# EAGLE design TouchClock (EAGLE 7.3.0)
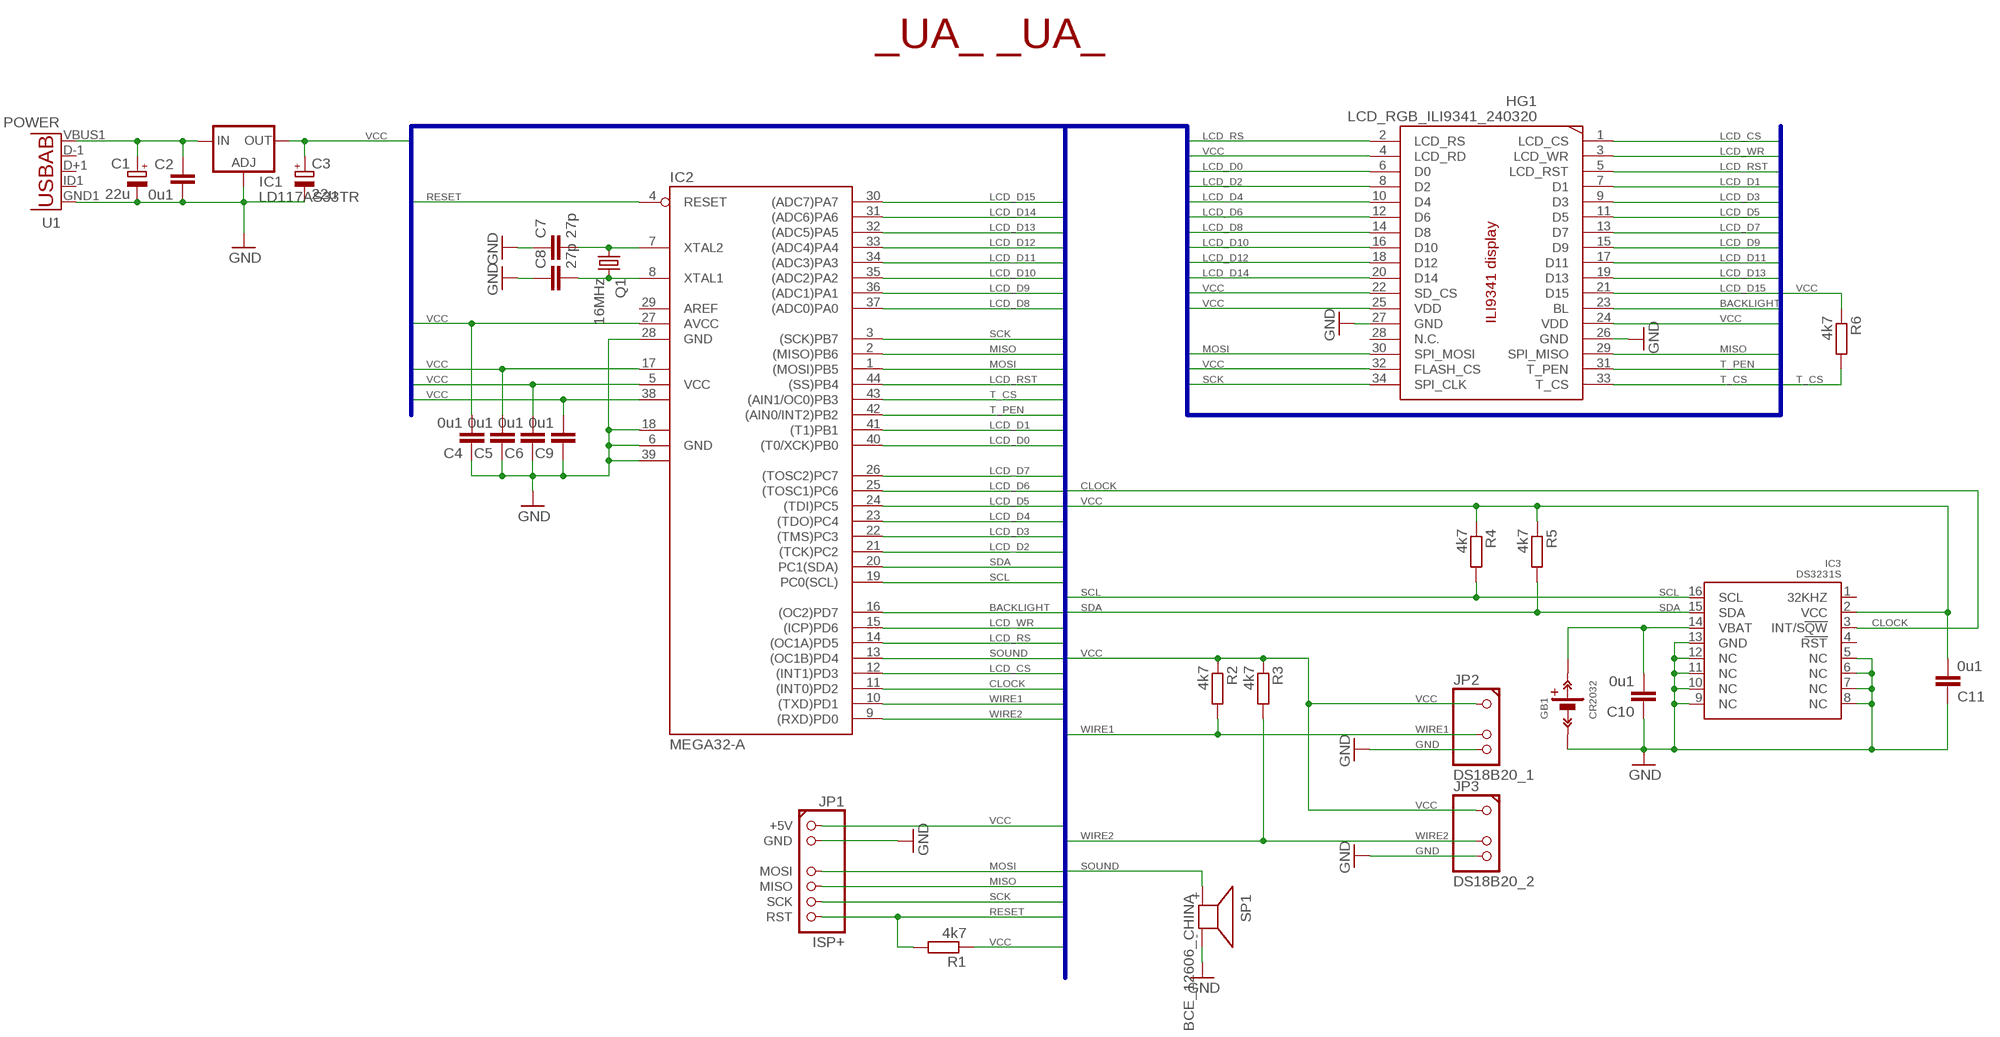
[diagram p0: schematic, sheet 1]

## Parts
C1  22u  CPOL-EUSMCB  [SMC_B]
C2  0u1  C-EUC1206T  [C1206T]
C3  22u  CPOL-EUSMCB  [SMC_B]
C4  0u1  C-EUC1206T  [C1206T]
C5  0u1  C-EUC1206T  [C1206T]
C6  0u1  C-EUC1206T  [C1206T]
C7  27p  C-EUC0805T  [C0805T]
C8  27p  C-EUC0805T  [C0805T]
C9  0u1  C-EUC1206T  [C1206T]
C10  0u1  C-EUC1206T  [C1206T]
C11  0u1  C-EUC1206T  [C1206T]
GB1  CR2032  CR2032_HOLDER/CH224  [CH224-2032]
HG1  LCD_RGB_ILI9341_240320  [2"4_320*240_ILI9341]
IC1  LD117AS33TR  [SOT223]
IC2  MEGA32-A  [TQFP44]
IC3  DS3231S  [SO16W]
JP1  ISP+  CONN1X7(2+4)_ISP+/R  [1X07_ISP+(ROUND)]
JP2  DS18B20_1  CONN1X4(1+2)/R90  [1X04ROUND/90(1+2)]
JP3  DS18B20_2  CONN1X4(1+2)/R90  [1X04ROUND/90(1+2)]
Q1  16MHz  CRYSTALHC49S  [HC49/S]
R1  4k7  R-EU_R0805T  [R0805T]
R2  4k7  R-EU_R0805T  [R0805T]
R3  4k7  R-EU_R0805T  [R0805T]
R4  4k7  R-EU_R0805T  [R0805T]
R5  4k7  R-EU_R0805T  [R0805T]
R6  4k7  R-EU_R0805T  [R0805T]
SP1  BCE_12606_CHINA  [BCE_12606_CHINA]
U1  POWER  USB5""  [USB-MICRO-SMD]
UA1  UA/MED  [UA_MED]
UA2  UA/SML  [UA_SMALL]

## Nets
BACKLIGHT: HG1.23(BL) IC2.16((OC2)PD7)
CLOCK: IC2.11((INT0)PD2) IC3.3(INT/SQW)
GND: C1.- C2.2 C3.- C4.1 C5.1 C6.1 C7.1 C8.1 C9.1 C10.1 C11.1 GB1.GB- HG1.26(GND) HG1.27(GND) IC1.1(ADJ) IC2.6(GND) IC2.18(GND1) IC2.28(GND) IC2.39(GND2) IC3.5(NC) IC3.6(NC) IC3.7(NC) IC3.8(NC) IC3.9(NC) IC3.10(NC) IC3.11(NC) IC3.12(NC) IC3.13(GND) JP1.GND JP2.4 JP3.4 SP1.- U1.GND1(GND)
LCD_CS: HG1.1(LCD_CS) IC2.12((INT1)PD3)
LCD_D0: HG1.6(D0) IC2.40((T0/XCK)PB0)
LCD_D1: HG1.7(D1) IC2.41((T1)PB1)
LCD_D2: HG1.8(D2) IC2.21((TCK)PC2)
LCD_D3: HG1.9(D3) IC2.22((TMS)PC3)
LCD_D4: HG1.10(D4) IC2.23((TDO)PC4)
LCD_D5: HG1.11(D5) IC2.24((TDI)PC5)
LCD_D6: HG1.12(D6) IC2.25((TOSC1)PC6)
LCD_D7: HG1.13(D7) IC2.26((TOSC2)PC7)
LCD_D8: HG1.14(D8) IC2.37((ADC0)PA0)
LCD_D9: HG1.15(D9) IC2.36((ADC1)PA1)
LCD_D10: HG1.16(D10) IC2.35((ADC2)PA2)
LCD_D11: HG1.17(D11) IC2.34((ADC3)PA3)
LCD_D12: HG1.18(D12) IC2.33((ADC4)PA4)
LCD_D13: HG1.19(D13) IC2.32((ADC5)PA5)
LCD_D14: HG1.20(D14) IC2.31((ADC6)PA6)
LCD_D15: HG1.21(D15) IC2.30((ADC7)PA7)
LCD_RS: HG1.2(LCD_RS) IC2.14((OC1A)PD5)
LCD_RST: HG1.5(LCD_RST) IC2.44((SS)PB4)
LCD_WR: HG1.3(LCD_WR) IC2.15((ICP)PD6)
MISO: HG1.29(SPI_MISO) IC2.2((MISO)PB6) JP1.MISO
MOSI: HG1.30(SPI_MOSI) IC2.1((MOSI)PB5) JP1.MOSI
N$1: C8.2 IC2.8(XTAL1) Q1.2
N$2: C7.2 IC2.7(XTAL2) Q1.1
N$5: C1.+ C2.1 IC1.3(IN) U1.VBUS1(VBUS)
RESET: IC2.4(RESET) JP1.RST R1.2
SCK: HG1.34(SPI_CLK) IC2.3((SCK)PB7) JP1.SCK
SCL: IC2.19(PC0(SCL)) IC3.16(SCL) R4.2
SDA: IC2.20(PC1(SDA)) IC3.15(SDA) R5.2
SOUND: IC2.13((OC1B)PD4) SP1.+
T_CS: HG1.33(T_CS) IC2.43((AIN1/OC0)PB3) R6.2
T_PEN: HG1.31(T_PEN) IC2.42((AIN0/INT2)PB2)
VBAT: C10.2 GB1.GB+ IC3.14(VBAT)
VCC: C3.+ C4.2 C5.2 C6.2 C9.2 C11.2 HG1.4(LCD_RD) HG1.22(SD_CS) HG1.24(VDD) HG1.25(VDD) HG1.32(FLASH_CS) IC1.4(OUT) IC2.5(VCC) IC2.17(VCC1) IC2.27(AVCC) IC2.38(VCC2) IC3.2(VCC) JP1.+5V JP2.1 JP3.1 R1.1 R2.1 R3.1 R4.1 R5.1 R6.1
WIRE1: IC2.10((TXD)PD1) JP2.3 R2.2
WIRE2: IC2.9((RXD)PD0) JP3.3 R3.2
Unconnected: HG1.28(N.C.) IC2.29(AREF) IC3.1(32KHZ) IC3.4(RST) U1.D+1(D+) U1.D-1(D-) U1.ID1(USBID)

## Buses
VCC,LCD_CS,LCD_WR,LCD_RST,LCD_RS,LCD_D[0..15],MISO,MOSI,SCK,T_PEN,T_CS,BACKLIGHT,RESET,SCL,SDA,WIRE1,WIRE2,CLOCK,SOUND

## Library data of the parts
C1 C3 = rcl:CPOL-EU: POLARIZED CAPACITOR, European symbol
C2 C4-C11 = rcl:C-EU: CAPACITOR, European symbol
GB1 = misc_passive_AL:CR2032_HOLDER: CR2032 Holder
HG1 = lcd-AL:LCD_RGB_ILI9341_240*320
IC1 = v-reg:LD117A?*: Low drop fixed and adjustable positive voltage regulators 1 A Source: http://www.st.com/stonline/products/literature/ds/7194/ld1117axx.pdf
IC2 = atmel:MEGA32: MICROCONTROLLER 32 Kbytes FLASH 2 Kbytes SRAM 1 Kbytes EEPROM USART 8-channel 10 bit ADC Source: www.atmel.com .. doc2503.pdf; MPN: ATMEGA32-16AU; OC_FARNELL: 9171274; OC_NEWARK: 69K6677
IC3 = misc-active-AL:DS3231S: TCXO Clock
JP1 = pinhead-AL:CONN1X7(2+4)_ISP+: PIN HEADER
JP2 JP3 = pinhead-AL:CONN1X4(1+2)
Q1 = crystal:CRYSTAL: CRYSTAL; OC_FARNELL: 1667008; OC_NEWARK: unknown
R1-R6 = rcl:R-EU_: RESISTOR, European symbol
SP1 = buzzer:BCE_12606_CHINA: BCE-12606
U1 = usb:USB5: This is a USB AB connector that is compatible with USB OTG. i.e. this connector can serve as a host or device
UA1 UA2 = misc_passive_AL:UA

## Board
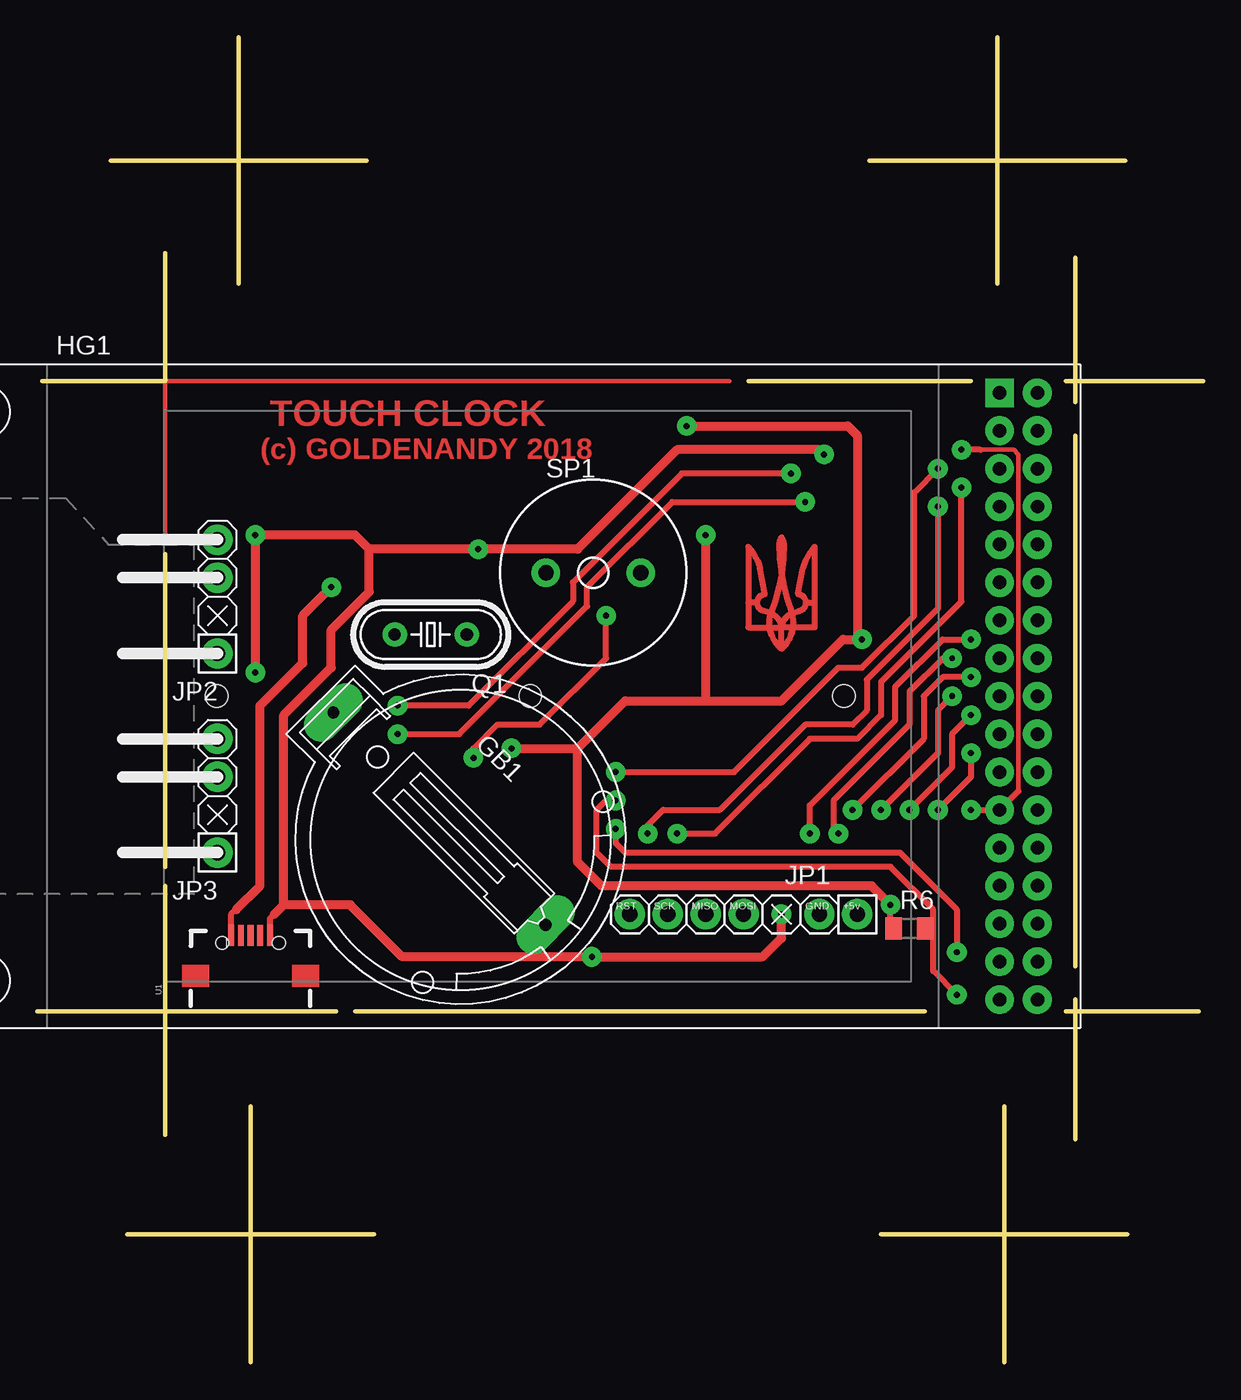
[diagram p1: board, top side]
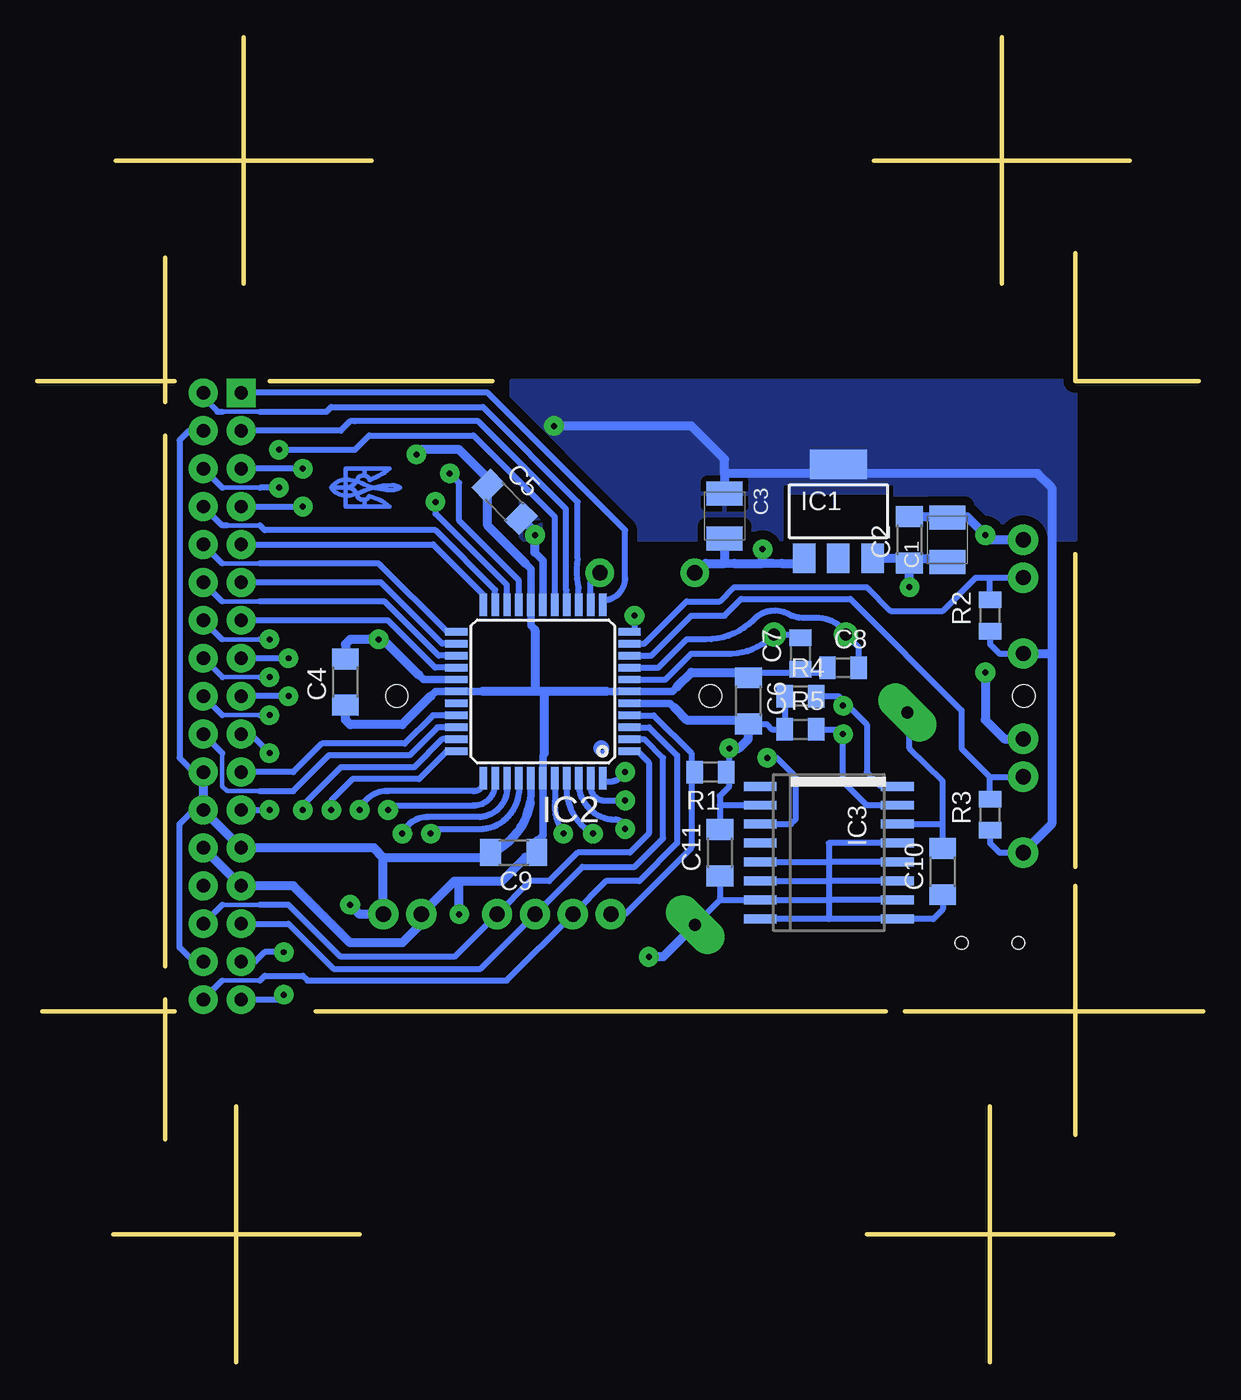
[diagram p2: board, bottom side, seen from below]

Size 78.11 x 88.74 mm. Coordinates in mm from the lower left corner, seen from the top.
Outline: 34 segments
Copper layers (1*16): Top 0.035mm / dielectric 1.5mm / Bottom 0.035mm
Design rules "default": minimum track width 12mil, minimum drill 10mil, track to track 10mil, track to pad 10mil, pad to pad 10mil, via to via 10mil, smd to smd 8mil, copper to edge 25mil, drill to drill 40mil, minimum pad ring 16mil, minimum via ring 18mil, stop-mask expansion 4mil, vias tented up to drill 0mil, thermal gap 16mil
Holes 1.5 mm at 54.02,44.61 33.02,44.61 12.02,44.61

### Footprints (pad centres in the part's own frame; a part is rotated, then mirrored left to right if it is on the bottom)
SMC_B = smd 1.6 x 2.4: + -1.5,0; - 1.5,0
C1206T = smd 1.4 x 1.8: 1 -1.55,0; 2 1.55,0
C0805T = smd 1.1 x 1.5: 1 -1.05,0; 2 1.05,0
CH224-2032 = drill 0.8 pad 2.3 long: GB+ -12.05,0; GB- 8.05,0
2"4_320*240_ILI9341 = drill 0.9 pad 1.93 square: 1 32.703,20.32 | drill 0.9 pad 1.93: 2 35.242,20.32; 3 32.703,17.78; 4 35.242,17.78; 5 32.703,15.24; 6 35.242,15.24; 7 32.703,12.7; 8 35.242,12.7; 9 32.703,10.16; 10 35.242,10.16; 11 32.703,7.62; 12 35.242,7.62; 13 32.703,5.08; 14 35.242,5.08; 15 32.703,2.54; 16 35.242,2.54; 17 32.703,0; 18 35.242,0; 19 32.703,-2.54; 20 35.242,-2.54; 21 32.703,-5.08; 22 35.242,-5.08; 23 32.703,-7.62; 24 35.242,-7.62; 25 32.703,-10.16; 26 35.242,-10.16; 27 32.703,-12.7; 28 35.242,-12.7; 29 32.703,-15.24; 30 35.242,-15.24; 31 32.703,-17.78; 32 35.242,-17.78; 33 32.703,-20.32; 34 35.242,-20.32
SOT223 = smd 1.5 x 2: 1 -2.3,-3.15; 2 0,-3.15; 3 2.3,-3.15 | smd 3.8 x 2: 4 0,3.15
TQFP44 = smd 1.5 x 0.5: 1 -5.8,4; 2 -5.8,3.2; 3 -5.8,2.4; 4 -5.8,1.6; 5 -5.8,0.8; 6 -5.8,0; 7 -5.8,-0.8; 8 -5.8,-1.6; 9 -5.8,-2.4; 10 -5.8,-3.2; 11 -5.8,-4; 23 5.8,-4; 24 5.8,-3.2; 25 5.8,-2.4; 26 5.8,-1.6; 27 5.8,-0.8; 28 5.8,0; 29 5.8,0.8; 30 5.8,1.6; 31 5.8,2.4; 32 5.8,3.2; 33 5.8,4 | smd 0.5 x 1.5: 12 -4,-5.8; 13 -3.2,-5.8; 14 -2.4,-5.8; 15 -1.6,-5.8; 16 -0.8,-5.8; 17 0,-5.8; 18 0.8,-5.8; 19 1.6,-5.8; 20 2.4,-5.8; 21 3.2,-5.8; 22 4,-5.8; 34 4,5.8; 35 3.2,5.8; 36 2.4,5.8; 37 1.6,5.8; 38 0.8,5.8; 39 0,5.8; 40 -0.8,5.8; 41 -1.6,5.8; 42 -2.4,5.8; 43 -3.2,5.8; 44 -4,5.8
SO16W = smd 0.6 x 2.2: 1 -4.445,-4.6; 2 -3.175,-4.6; 3 -1.905,-4.6; 4 -0.635,-4.6; 5 0.635,-4.6; 6 1.905,-4.6; 7 3.175,-4.6; 8 4.445,-4.6; 9 4.445,4.6; 10 3.175,4.6; 11 1.905,4.6; 12 0.635,4.6; 13 -0.635,4.6; 14 -1.905,4.6; 15 -3.175,4.6; 16 -4.445,4.6
1X07_ISP+(ROUND) = drill 1.016 pad 2.032: +5V -7.62,0; GND -5.08,0; MISO 2.54,0; MOSI 0,0; RST 7.62,0; SCK 5.08,0
1X04ROUND/90(1+2) = drill 1.016 pad 2.032: 1 -3.81,0; 3 1.27,0; 4 3.81,0
HC49/S = drill 0.813: 1 -2.413,0; 2 2.413,0
R0805T = smd 1.1 x 1.5: 1 -1.05,0; 2 1.05,0
BCE_12606_CHINA = drill 1.016 pad 1.905: + 3.175,0; - -3.175,0
USB-MICRO-SMD = smd 1.4 x 0.4: D+1 2.7,0; D-1 2.7,0.65; GND1 2.7,-1.3; ID1 2.7,-0.65; VBUS1 2.7,1.3 | hole 0.85: 2.2,1.9; 2.2,-1.9

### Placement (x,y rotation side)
C1  17.14,55.09 90 bottom
C2  19.69,55.09 90 bottom
C3  32.07,56.67 270 bottom
C4  57.47,45.56 90 bottom
C5  46.8,57.63 315 bottom
C6  30.48,44.29 270 bottom
C7  26.99,47.47 90 bottom
C8  24.13,46.51 0 bottom
C9  46.2,34.13 180 bottom
C10  17.46,32.86 90 bottom
C11  32.38,34.13 90 bottom
GB1  28.35,34.99 315 top
HG1  31.75,44.61 0 top
IC1  24.45,56.99 0 bottom
IC2  44.24,44.93 180 bottom
IC3  25.08,34.13 270 bottom
JP1  47.31,30 180 top
JP2  12.06,51.28 90 top
JP3  12.06,37.94 90 top
Q1  26.35,48.74 180 top
R1  33.02,39.53 180 bottom
R2  14.29,50.01 90 bottom
R3  14.29,36.67 90 bottom
R4  26.99,44.61 0 bottom
R5  26.99,42.39 0 bottom
R6  58.42,29.05 0 top
SP1  37.24,52.88 0 top
U1  14.29,25.88 90 top
UA1  49.85,51.28 0 top
UA2  56.52,58.58 270 bottom

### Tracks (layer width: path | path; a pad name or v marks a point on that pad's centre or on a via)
BACKLIGHT  (via drill 0.4)
  Top 0.305: 65.72,38.26 65.72,60.8 65.41,61.12 63.18,61.12
  Top 0.406: v62.55,36.99 HG1.23 65.72,38.26 | 63.18,61.12 v61.91,61.12
  Bottom 0.406: HG1.23 v62.55,36.99 | v61.91,61.12 56.83,61.12 55.88,62.07 48.9,62.07 43.44,56.62 IC2.16
CLOCK  (via drill 0.4)
  Top 0.406: v29.21,40.48 29.21,41.12 30.8,42.7 33.66,42.7 38.1,47.15 v38.1,50.01
  Bottom 0.406: IC3.3 27.62,36.04 27.3,36.35 27.3,39.21 28.58,40.48 v29.21,40.48 | v38.1,50.01 38.1,49.05 38.23,48.93 IC2.11
GND  (via drill 0.4)
  Top 0.406: U1.GND1 15.59,29.72 15.87,30
  Top 0.61: v49.85,30 49.85,28.42 48.58,27.15 v37.15,27.15 24.45,27.15 20.95,30.64 16.51,30.64 | 15.87,30 16.51,30.64 | 16.51,30.64 16.51,43.34 19.69,46.51 19.69,49.05 22.23,51.59 22.23,54.45 | v52.7,60.8 52.39,61.12 42.86,61.12 36.2,54.45 v29.53,54.45 22.23,54.45 | 22.23,54.45 21.27,55.4 v14.6,55.4 v14.6,46.2
  Bottom 0.406: 40.01,44.93 | 48.26,44.93 | C6.1 30.52,46.2 26.99,46.2 | 26.99,46.2 25.5,46.2 C8.1 | C7.1 26.99,46.2 | 25.08,29.69 IC3.9 18.1,29.69 17.46,30.32 C10.1 | 25.08,29.69 IC3.8 | IC3.10 25.08,30.96 | 25.08,30.96 25.08,29.69 | IC3.11 25.08,32.23 | 25.08,32.23 25.08,30.96 | IC3.12 25.08,33.5 | 25.08,33.5 25.08,32.23 | IC3.13 25.08,34.77 25.08,33.5 | 25.08,30.96 IC3.7 32.38,30.96 | IC3.6 25.08,32.23 | IC3.5 25.08,33.5 | GB1.GB- | GB1.GB- 32.38,30.96 | C11.1 32.38,30.96
  Bottom 0.508: 44.13,40.8 44.24,40.59 IC2.39 44.24,35.29 44.61,34.92 | 40.01,44.93 IC2.6 35.56,44.93 35.24,45.24 | 48.26,44.93 IC2.28 51.44,44.93 51.75,44.61 | 44.77,49.05 45.04,49.33 IC2.18 45.04,53.14 45.4,53.5
  Bottom 0.61: HG1.26 HG1.27 60.96,31.91 57.15,28.1 53.66,28.1 52.39,29.37 JP1.GND 50.17,32.23 49.85,32.23 | 44.77,49.05 44.77,44.93 | 44.77,44.93 48.26,44.93 | 40.01,44.93 44.13,44.93 | 44.13,44.93 44.77,44.93 | 44.13,40.8 44.13,44.93 | 35.24,45.24 34.29,46.2 30.52,46.2 | 45.4,53.5 47.94,56.04 47.94,58.68 C5.1 47.9,59.17 49.85,61.12 52.39,61.12 v52.7,60.8 | 44.61,34.92 44.77,34.77 44.77,33.81 | 44.77,33.81 45.4,33.81 46.99,32.23 49.85,32.23 | C9.1 44.77,33.81 | v49.85,30 49.85,32.23 | GB1.GB- | GB1.GB- 36.2,27.15 v37.15,27.15 | SP1.- 33.34,53.5 32.08,53.5 32.07,53.51 | C3.- 32.07,53.51 | 32.07,53.51 31.43,53.5 29.55,53.5 29.53,53.51 | 29.53,53.51 28.88,53.51 28.26,53.5 26.77,53.5 IC1.1 | 29.53,53.51 29.53,54.13 v29.53,54.45 | JP2.4 14.29,55.09 v14.6,55.4 15.84,56.64 17.14,56.64 | v14.6,46.2 14.6,43.02 13.33,41.75 JP3.4 | C2.2 17.14,56.64 | C1.- 17.14,56.64 | 51.75,44.61 53.66,42.7 57.15,42.7 57.47,43.02 C4.1
LCD_CS
  Bottom 0.406: HG1.1 47.94,64.93 38.73,55.72 38.73,52.55 arc93 40.24,51.04 IC2.12
LCD_D0  (via drill 0.4)
  Top 0.406: v42.86,35.4 45.4,35.4 51.75,41.75 54.93,41.75 56.52,43.34 56.52,45.56 61.91,50.96 v61.91,58.58
  Bottom 0.305: 63.18,58.58 65.72,58.58
  Bottom 0.406: IC2.40 43.44,37.57 arc-38 v42.86,35.4 | v61.91,58.58 63.18,58.58 | 65.72,58.58 HG1.6
LCD_D1  (via drill 0.4)
  Top 0.406: v40.88,35.4 40.88,35.96 41.91,36.99 45.72,36.99 51.44,42.7 54.61,42.7 55.56,43.66 55.56,45.72 60.33,50.48 v60.33,57.31
  Bottom 0.406: IC2.41 42.64,38.04 arc-54 v40.88,35.4 | HG1.7 v60.33,57.31
LCD_D2
  Bottom 0.305: 63.18,56.04 65.41,56.04
  Bottom 0.406: IC2.21 47.44,51.73 51.44,55.72 62.86,55.72 63.18,56.04 | 65.41,56.04 65.72,56.04 HG1.8
LCD_D3
  Bottom 0.406: HG1.9 51.59,54.77 48.24,51.42 IC2.22
LCD_D4
  Bottom 0.305: 65.72,53.5 63.18,53.5
  Bottom 0.406: HG1.10 65.72,53.5 | IC2.23 50.67,48.93 55.25,53.5 63.18,53.5
LCD_D5
  Bottom 0.406: IC2.24 50.98,48.13 55.09,52.23 HG1.11
LCD_D6
  Bottom 0.305: 65.72,50.96 63.18,50.96
  Bottom 0.406: HG1.12 65.72,50.96 | IC2.25 51.22,47.33 54.85,50.96 63.18,50.96
LCD_D7
  Bottom 0.406: IC2.26 51.45,46.53 54.61,49.69 HG1.13
LCD_D8  (via drill 0.4)
  Top 0.406: v51.75,35.4 51.75,37.31 57.47,43.02 57.47,45.24 60.64,48.42 v62.55,48.42
  Bottom 0.305: 65.72,48.42 63.18,48.42
  Bottom 0.406: HG1.14 65.72,48.42 | 63.18,48.42 v62.55,48.42 | IC2.37 45.84,38.14 arc79 48.26,35.72 51.44,35.72 v51.75,35.4
LCD_D9  (via drill 0.4)
  Top 0.406: v61.28,47.15 60.64,47.15 58.42,44.93 58.42,42.7 53.34,37.62 53.34,35.72 v53.66,35.4
  Bottom 0.406: IC2.36 46.64,38.29 arc79 48.42,36.51 51.91,36.51 arc-67 v53.66,35.4 | v61.28,47.15 HG1.15
LCD_D10  (via drill 0.4)
  Top 0.406: v62.55,45.88 60.64,45.88 59.37,44.61 59.37,41.75 v54.61,36.99
  Bottom 0.305: 65.72,45.88 63.18,45.88
  Bottom 0.406: HG1.16 65.72,45.88 | 63.18,45.88 v62.55,45.88 | v54.61,36.99 54.29,37.31 48.9,37.31 arc-96 47.44,38.76 IC2.35
LCD_D11  (via drill 0.4)
  Top 0.406: v61.28,44.61 60.33,43.66 60.33,40.8 v56.52,36.99
  Bottom 0.406: IC2.34 48.24,38.91 arc104 48.9,38.26 54.61,38.26 arc-70 v56.52,36.99 | v61.28,44.61 HG1.17
LCD_D12  (via drill 0.4)
  Top 0.406: v62.55,43.34 61.28,42.07 61.28,39.85 v58.42,36.99
  Bottom 0.305: 65.72,43.34 63.18,43.34
  Bottom 0.406: HG1.18 65.72,43.34 | 63.18,43.34 v62.55,43.34 | IC2.33 50.67,40.93 52.55,39.05 56.99,39.05 58.42,37.62 v58.42,36.99
LCD_D13  (via drill 0.4)
  Top 0.406: v62.55,40.8 62.55,39.21 v60.33,36.99
  Bottom 0.406: v60.33,36.99 60.33,37.31 57.78,39.85 52.86,39.85 50.98,41.73 IC2.32 | v62.55,40.8 63.82,42.07 HG1.19
LCD_D14
  Bottom 0.305: 65.72,40.8 65.72,38.58 65.41,38.26 63.18,38.26
  Bottom 0.406: HG1.20 65.72,40.8 | 63.18,38.26 60.96,38.26 58.58,40.64 53.18,40.64 51.3,42.53 IC2.31
LCD_D15
  Bottom 0.406: HG1.21 60.96,39.53 59.06,41.43 53.5,41.43 51.61,43.33 IC2.30
LCD_RS
  Bottom 0.305: 65.72,63.66 63.18,63.66
  Bottom 0.406: HG1.2 66.99,64.61 66.04,63.66 65.72,63.66 | 63.18,63.66 58.74,63.66 58.42,63.98 48.26,63.98 41.91,57.63 41.91,53.82 arc-19 41.91,52.15 41.84,51.84 IC2.14
LCD_RST  (via drill 0.4)
  Top 0.406: v38.73,39.53 46.67,39.53 53.66,46.51 55.25,46.51 58.74,50.01 58.74,58.26 v60.33,59.85
  Bottom 0.406: IC2.44 40.24,38.81 40.01,38.89 39.69,38.89 arc-56 v38.73,39.53 | v60.33,59.85 HG1.5
LCD_WR
  Bottom 0.406: HG1.3 57.78,62.39 57.15,63.02 56.83,63.02 48.58,63.02 42.7,57.15 42.7,51.75 42.64,51.69 IC2.15
MISO
  Bottom 0.406: IC2.2 37.44,41.73 36.2,40.48 36.2,35.08 38.1,33.18 41.59,33.18 JP1.MISO 48.42,26.35 58.26,26.35 61.28,29.37 HG1.29
MOSI
  Bottom 0.305: 63.18,30.64 65.72,30.64
  Bottom 0.406: IC2.1 37.91,40.93 37.15,40.16 37.15,35.4 38.42,34.13 41.91,34.13 43.81,32.23 45.09,32.23 JP1.MOSI 50.17,27.15 57.78,27.15 61.28,30.64 63.18,30.64 | 65.72,30.64 HG1.30
N$1
  Bottom 0.406: C8.2 23.08,47.88 Q1.2 23.94,48.86 arc-50 25.72,49.85 26.67,49.85 arc21 27.62,50.01 arc-81 30.16,49.69 arc45 33.34,48.42 34.61,48.42 36.5,46.53 IC2.8
N$2
  Bottom 0.406: IC2.7 36.03,45.73 34.29,47.47 31.94,47.47 arc-48 Q1.1 27.21,48.74 C7.2
N$3
  Top 0.305: 8.57,55.09 8.57,65.72 46.36,65.72
N$5  (via drill 0.4)
  Top 0.406: U1.VBUS1 12.99,30.03 13.33,30.32
  Top 0.61: 13.33,30.32 14.92,31.91 14.92,43.97 17.78,46.83 17.78,50.01 v19.69,51.91
  Bottom 0.61: v19.69,51.91 C2.1 19.69,53.82 | 19.69,53.82 21.86,53.82 IC1.3 | 19.69,53.82 17.55,53.82 C1.+
RESET
  Bottom 0.406: IC2.4 36.82,43.33 34.29,40.8 34.29,39.53 | 34.29,39.53 34.29,34.45 38.73,30 JP1.RST | R1.2 34.29,39.53
SCK
  Bottom 0.305: 65.72,25.56 63.18,25.56
  Bottom 0.406: IC2.3 37.13,42.53 35.24,40.64 35.24,34.77 37.78,32.23 40.01,32.23 JP1.SCK 46.67,25.56 60.01,25.56 60.33,25.88 62.86,25.88 63.18,25.56 | HG1.34 65.72,25.56
SCL  (via drill 0.4)
  Top 0.406: v50.48,59.53 43.18,59.53 35.88,52.23 35.88,50.96 28.89,43.97 v24.13,43.97
  Bottom 0.406: IC2.19 45.84,52.35 49.85,56.36 49.85,58.9 v50.48,59.53 | v24.13,43.97 23.81,43.97 | 23.81,43.97 22.54,42.7 22.54,39.53 21.59,38.58 IC3.16 | R4.2 24.45,44.61 23.81,43.97
SDA  (via drill 0.4)
  Top 0.406: v24.13,42.07 28.26,42.07 36.83,50.64 36.83,51.91 42.55,57.63 v51.44,57.63
  Bottom 0.406: IC3.15 22.54,37.31 24.13,38.89 v24.13,42.07 24.45,42.39 R5.2 | v51.44,57.63 51.44,56.83 46.64,52.04 IC2.20
SOUND
  Bottom 0.406: IC2.13 41.04,52.25 SP1.+
T_CS  (via drill 0.4)
  Top 0.406: v61.59,24.61 60.01,26.19 60.01,29.05 | 60.01,29.05 60.01,30.32 57.15,33.18 38.42,33.18 37.47,34.13 37.47,36.99 38.1,37.62 v38.73,37.62 | R6.2 60.01,29.05
  Bottom 0.406: IC2.43 41.04,38.66 arc-102 40.01,37.62 v38.73,37.62 | HG1.33 61.91,24.29 v61.59,24.61
T_PEN  (via drill 0.4)
  Top 0.406: v38.73,35.72 38.73,34.77 39.37,34.13 57.78,34.13 61.59,30.32 v61.59,27.46
  Bottom 0.406: IC2.42 41.84,38.51 arc-75 39.69,36.35 39.37,36.35 arc83 v38.73,35.72 | v61.59,27.46 62.86,27.46 63.5,26.83 HG1.31
VBAT
  Bottom 0.406: IC3.14 17.46,36.04 | 17.46,36.04 17.46,38.92 19.69,41.12 19.69,43.37 GB1.GB+ | C10.2 17.46,36.04
VCC  (via drill 0.4)
  Top 0.406: R6.1 57.15,29.05 v57.15,30.64
  Top 0.61: 36.2,41.12 39.37,44.29 44.77,44.29 | 44.77,44.29 49.85,44.29 53.97,48.42 v55.25,48.42 54.93,48.42 54.93,62.07 54.29,62.71 v43.5,62.71 | v44.77,55.4 44.77,44.29 | v57.15,30.64 55.88,31.91 37.78,31.91 36.2,33.5 36.2,41.12 | v31.75,41.12 36.2,41.12
  Bottom 0.406: HG1.4 67.95,62.39 68.58,61.75 68.58,40.48 67.63,39.53 HG1.22 | HG1.32 67.63,26.83 68.58,27.78 68.58,36.04 67.63,36.99 HG1.24 | 30.52,43.02 C6.2 29.25,42.74 28.89,42.39 R5.1 R4.1 | 32.38,37.31 32.38,37.94 31.75,38.58 31.75,39.53 | 32.38,37.31 C11.2 | IC3.2 32.38,37.31 | R3.1 14.29,34.77 13.65,34.13 JP3.1 | R2.1 14.29,48.1 13.65,47.47 JP2.1 | 31.75,39.53 v31.75,41.12 | R1.1 31.75,39.53
  Bottom 0.508: IC2.5 35.73,44.13 35.41,43.82 | IC2.17 44.24,53.71 44.77,54.23 | IC2.38 45.04,37.98 45.09,37.46 | IC2.27 52.23,45.73 52.55,46.04
  Bottom 0.61: HG1.22 HG1.24 HG1.25 55.56,34.45 54.93,33.81 | 35.41,43.82 34.61,43.02 30.52,43.02 | 52.55,46.04 54.93,48.42 v55.25,48.42 57.15,48.42 57.47,48.1 C4.2 | 44.77,54.23 v44.77,55.4 44.77,55.59 C5.2 | 54.93,33.81 JP1.+5V 56.52,30 v57.15,30.64 | 54.93,33.81 48.26,33.81 47.94,34.13 C9.2 47.62,34.13 arc-53 45.09,37.46 | 24.42,59.85 IC1.4 24.45,59.53 | 32.07,59.53 32.07,60.48 34.29,62.71 v43.5,62.71 | 24.45,59.53 11.11,59.53 10.16,58.58 10.16,47.47 | 24.45,59.53 32.07,59.53 | 32.07,59.53 C3.+ | 10.16,47.47 10.16,36.04 JP3.1 | JP2.1 10.16,47.47 | v31.75,41.12 31.12,41.12 30.48,41.75 C6.2
  pour Bottom (isolate 0.61, no thermals): 22.23,58.26 27.62,58.26 27.62,62.07 21.27,62.07 21.27,58.26
  pour Bottom (isolate 0.61): 20.64,58.9 20.64,55.09 8.57,55.09 8.57,65.72 46.36,65.72 46.36,55.09 28.26,55.09 28.26,58.9
WIRE1
  Bottom 0.406: IC2.10 37.44,48.13 34.61,50.96 32.38,50.96 31.43,51.91 22.54,51.91 20.95,50.32 17.46,50.32 15.24,52.55 14.29,52.55 | 14.29,52.55 JP2.3 | R2.2 14.29,52.55
WIRE2
  Bottom 0.406: IC2.9 36.97,47.33 34.29,50.01 32.07,50.01 30.96,51.12 23.65,51.12 16.19,43.66 16.19,41.12 14.29,39.21 | 14.29,39.21 JP3.3 | R3.2 14.29,39.21
(copper drawn outside any net)
  shapes: Bottom circle x1

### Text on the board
Top: TOUCH CLOCK | (c) GOLDENANDY 2018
